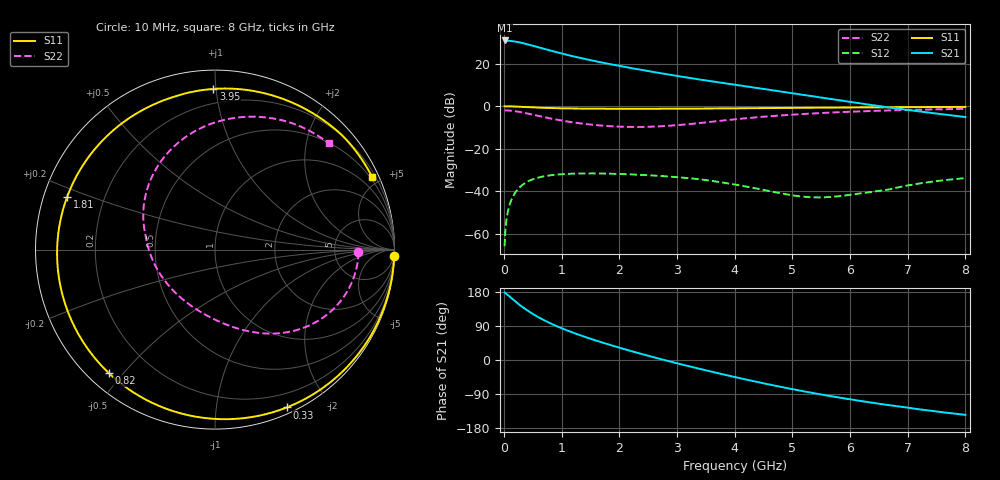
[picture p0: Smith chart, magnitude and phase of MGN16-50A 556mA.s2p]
! Port[1] = GATE
! Port[2] = DRAIN
! [Type]  S-parameter s2p file touchstone ver. 1.0
! [Object]  MGN16-50A
! [Bias]  556 mA
! [Version]  1.0
! [Date]  Thu May 28 11:05:48 2026
! [Source]  This file was created in JSC "ICC Milandr".
! [Disclaimer] Property of JSC "ICC Milandr". Unauthorized reproduction and/or distribution is strictly prohibited.
!  The file and the data are provided "AS IS" and with all faults and disclaim all warranties, express and implied, including
!  without limitation any implied warranties of merchantability, fitness for a particular purpose.
!  JSC "ICC Milandr" assumes no liability for:
!  1) the accuracy of the data provided;
!  2) the proper functioning of this data;
!  3) infringement of patents, copyrights or intellectual property rights resulting from the use of this data.
!  JSC "ICC Milandr" reserves the right to make changes to the products and the data without prior notice.
!  Please, be aware that your receipt and use of the file provided shall serve as acceptance of these terms and conditions.
!  If you do not accept these terms, you should return or destroy this file and any other accompanying information immediately.
# hz S ma R 12.5
! 2 Port Network Data from SP1.SP block
! freq  magS11  angS11  magS21  angS21  magS12  angS12  magS22  angS22
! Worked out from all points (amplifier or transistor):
!   800 points, 10 MHz to 8 GHz, reference 12.5 ohm
!   highest |S21| = 30.9 dB at 10 MHz (marker M1)
!   |S21| within 3 dB of that: start of sweep to 570.4 MHz
!   unconditionally stable (mu >= 1): 3.696 GHz to 7.317 GHz
!   at 1.34 GHz: K = 0.23, MSG = 27.1 dB, |S12| = -31.6 dB
!   at 4.01 GHz: K = 1.21, MAG = 20.7 dB, |S12| = -36.8 dB
!   at 8 GHz: K = 0.72, MSG = 14.4 dB, |S12| = -33.8 dB
!   S11 on the Smith chart (normalised r, x): 10 MHz: 2, -54; 330 MHz: 0.06, -1.55; 820 MHz: 0.06, -0.46; 1.81 GHz: 0.07, +0.17; 3.95 GHz: 0.11, +0.98; 8 GHz: 0.38, +4.50
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1e7  0.9988 -2.1  35.25 178.5  0.0005142 80.7  0.7994 -1.0
4e7  0.9983 -8.6  35.06 174.5  0.002026 82.8  0.7983 -4.3
8e7  0.9964 -17.0  34.78 169.2  0.004019 78.7  0.7936 -8.5
1.5e8  0.9905 -31.5  33.95 160.1  0.00736 70.5  0.7781 -15.7
2.4e8  0.9793 -49.2  32.37 149.0  0.01124 60.1  0.7477 -24.4
3.3e8  0.966 -65.5  30.44 138.7  0.01454 50.4  0.71 -32.4
4.2e8  0.9525 -80.4  28.36 129.2  0.01726 41.5  0.6695 -39.6
5.3e8  0.9371 -96.6  25.84 118.7  0.01987 31.7  0.6206 -47.4
6.7e8  0.9207 -114.5  22.89 106.9  0.02226 20.7  0.5638 -56.1
8.2e8  0.9072 -130.8  20.14 95.7  0.02399 10.5  0.5118 -64.3
1.06e9  0.8924 -152.4  16.6 80.1  0.02557 -3.7  0.4469 -76.1
1.35e9  0.8821 -173.4  13.42 63.8  0.02632 -18.4  0.3923 -89.4
1.56e9  0.8777 173.9  11.65 53.0  0.02637 -27.9  0.3647 -99.2
1.81e9  0.8747 160.6  9.956 41.1  0.02608 -38.5  0.3422 -111.4
2.23e9  0.8729 141.7  7.8 22.5  0.02496 -55.1  0.3262 -133.4
2.68e9  0.8744 124.9  6.115 3.9  0.02313 -71.8  0.3367 -158.1
3.25e9  0.8803 107.5  4.557 -18.1  0.02015 -91.8  0.3853 172.3
3.95e9  0.8952 90.6  3.295 -43.2  0.0149 -102.8  0.4861 143.3
4.01e9  0.8965 89.3  3.205 -45.3  0.01443 -103.3  0.4951 141.0
5.34e9  0.9241 63.1  1.72 -86.7  0.007238 -80.6  0.6763 97.9
6.67e9  0.952 42.4  0.9381 -118.9  0.01102 -50.7  0.7982 66.4
8e9  0.9648 24.9  0.5579 -144.8  0.02047 -59.5  0.8674 43.0
